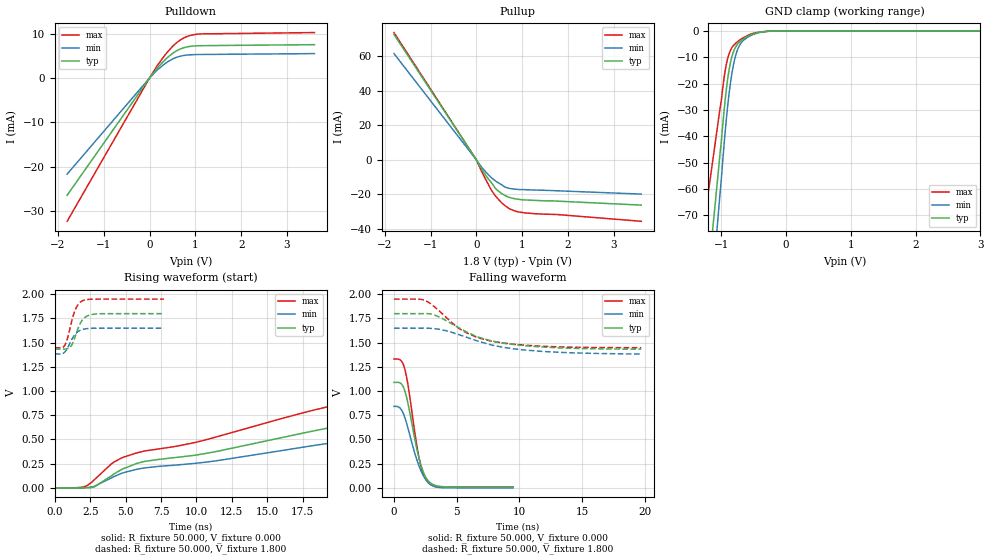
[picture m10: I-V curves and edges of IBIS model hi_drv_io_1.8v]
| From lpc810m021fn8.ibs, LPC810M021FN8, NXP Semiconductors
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[Model]   hi_drv_io_1.8v
Model_type I/O
Vinl=5.400E-01
Vinh=1.260E+00
Vref=0.000E+00
Rref=1.000E+06
Cref=2.000E-11
Vmeas=9.000E-01
C_comp   8.440E-13   8.280E-13   8.600E-13
[Voltage Range]   1.800E+00   1.650E+00   1.950E+00
[POWER Clamp Reference]   1.800E+00   1.650E+00   1.950E+00
[GND Clamp Reference]   0.000E+00   0.000E+00   0.000E+00
[Pullup Reference]   1.800E+00   1.650E+00   1.950E+00
[Pulldown Reference]   0.000E+00   0.000E+00   0.000E+00
[Temperature Range]   25   85   -40
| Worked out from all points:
|   slope of the pulldown table from 0 to 0.27 V, typ, clamps not added: 80.1 ohm
|   slope of the pullup table from 0 to 0.27 V, typ, clamps not added: 23.9 ohm
|   GND clamp passes 1 mA (typ) near -0.49 V on its own axis
|   rising waveform, R_fixture 50.000, V_fixture 0.000: 20-80 % time 25.4ns typ, 27ns min, 22.9ns max; typ from 0 V to 1.08 V
|   falling waveform, R_fixture 50.000, V_fixture 0.000: 20-80 % time 1.06ns typ, 1.19ns min, 948ps max; typ from 1.09 V to 0.008 V
|   rising waveform, R_fixture 50.000, V_fixture 1.800: 20-80 % time 612ps typ, 623ps min, 573ps max; typ from 1.43 V to 1.8 V
|   falling waveform, R_fixture 50.000, V_fixture 1.800: 20-80 % time 4.03ns typ, 4.67ns min, 3.37ns max; typ from 1.8 V to 1.43 V
[GND Clamp]
-1.8V     -244.7mA   -289.3mA   -167mA
-1.02V    -46.52mA   -61.63mA   -29.35mA
-960mV    -30.82mA   -43.78mA   -18.18mA
-920mV    -21.59mA   -32.78mA   -12.28mA
-880mV    -14.7mA    -23.66mA   -8.632mA
-840mV    -10.06mA   -16.55mA   -6.501mA
-800mV    -7.146mA   -11.36mA   -5.216mA
-760mV    -5.376mA   -7.82mA    -4.319mA
-660mV    -3.02mA    -3.637mA   -2.604mA
-440mV    -697.2uA   -814.9uA   -584.6uA
-100mV    -9.428uA   -9.367uA   -9.062uA
3.6V      0A         0A         0A
[POWER Clamp]
-1.8V     0A         0A         0A
3.6V      0A         0A         0A
[Pullup]
-1.8V     72.63mA    61.52mA    73.68mA
0V        0A         0A         0A
120mV     -5.537mA   -4.377mA   -6.97mA
340mV     -13.63mA   -10.59mA   -18.06mA
440mV     -17.14mA   -12.62mA   -21.6mA
620mV     -20.57mA   -15.66mA   -26.4mA
720mV     -21.71mA   -16.48mA   -28.23mA
820mV     -22.4mA    -16.9mA    -29.37mA
1.06V     -23.19mA   -17.26mA   -30.69mA
1.78V     -23.9mA    -17.91mA   -31.67mA
3.6V      -26.18mA   -19.81mA   -35.55mA
[Pulldown]
-1.8V     -26.45mA   -21.68mA   -32.33mA
0V        0A         0A         0A
140mV     1.894mA    1.524mA    2.352mA
320mV     3.921mA    3.1mA      4.945mA
500mV     5.53mA     4.273mA    7.104mA
600mV     6.19mA     4.713mA    8.047mA
740mV     6.8mA      5.071mA    8.997mA
880mV     7.124mA    5.228mA    9.584mA
1.14V     7.298mA    5.309mA    9.953mA
3.6V      7.517mA    5.502mA    10.25mA
[Rising Waveform]
R_fixture = 50.000
V_fixture = 0.000
V_fixture_min = 0.000
V_fixture_max = 0.000
|  time   V(typ)   V(min)   V(max)
0s        0V         0V         0V
2.2ns     322.1uV    1.74mV     17.8mV
2.8ns     10.34mV    16.3mV     84.91mV
4.2ns     145.5mV    117.9mV    268.4mV
5.8ns     253.2mV    192.5mV    362mV
10ns      339.9mV    255mV      472.4mV
20.3ns    646.8mV    481.9mV    874.3mV
27.2ns    807.9mV    608mV      1.062V
44.5ns    1.017V     777.6mV    1.273V
62.9ns    1.084V     842.5mV    1.325V
[Falling Waveform]
R_fixture = 50.000
V_fixture = 0.000
V_fixture_min = 0.000
V_fixture_max = 0.000
|  time   V(typ)   V(min)   V(max)
0s        1.09V      842.5mV    1.332V
600ps     1.073V     806.3mV    1.31V
900ps     988.4mV    713.9mV    1.21V
1.1ns     882.7mV    624.7mV    1.077V
1.7ns     480.3mV    340.5mV    537.9mV
2ns       306.5mV    225.1mV    309.2mV
2.3ns     176.9mV    136.8mV    156.7mV
2.7ns     77.06mV    59.55mV    58.17mV
3.9ns     12mV       1.329mV    7.864mV
9.5ns     7.852mV    0V         8.054mV
[Rising Waveform]
R_fixture = 50.000
V_fixture = 1.800
V_fixture_min = 1.650
V_fixture_max = 1.950
|  time   V(typ)   V(min)   V(max)
0s        1.433V     1.384V     1.448V
700ps     1.434V     1.402V     1.471V
900ps     1.438V     1.444V     1.545V
1.1ns     1.456V     1.504V     1.664V
1.3ns     1.507V     1.559V     1.778V
1.5ns     1.589V     1.598V     1.857V
1.8ns     1.7V       1.628V     1.918V
2ns       1.744V     1.638V     1.936V
3ns       1.798V     1.65V      1.95V
7.7ns     1.8V       1.65V      1.95V
[Falling Waveform]
R_fixture = 50.000
V_fixture = 1.800
V_fixture_min = 1.650
V_fixture_max = 1.950
|  time   V(typ)   V(min)   V(max)
0s        1.8V       1.65V      1.95V
2ns       1.8V       1.65V      1.949V
2.5ns     1.801V     1.65V      1.934V
3.6ns     1.766V     1.639V     1.829V
5.4ns     1.637V     1.573V     1.629V
6.5ns     1.568V     1.524V     1.561V
7.6ns     1.524V     1.482V     1.52V
9.5ns     1.482V     1.437V     1.484V
11.9ns    1.455V     1.409V     1.462V
19.7ns    1.433V     1.384V     1.448V
[Ramp]
dV/dt_r   6.4905E-01/2.5463E-08   5.0919E-01/2.6995E-08   7.9413E-01/2.2932E-08
dV/dt_f   2.2020E-01/4.0258E-09   1.5981E-01/4.6723E-09   3.0112E-01/3.3613E-09
R_load = 50
